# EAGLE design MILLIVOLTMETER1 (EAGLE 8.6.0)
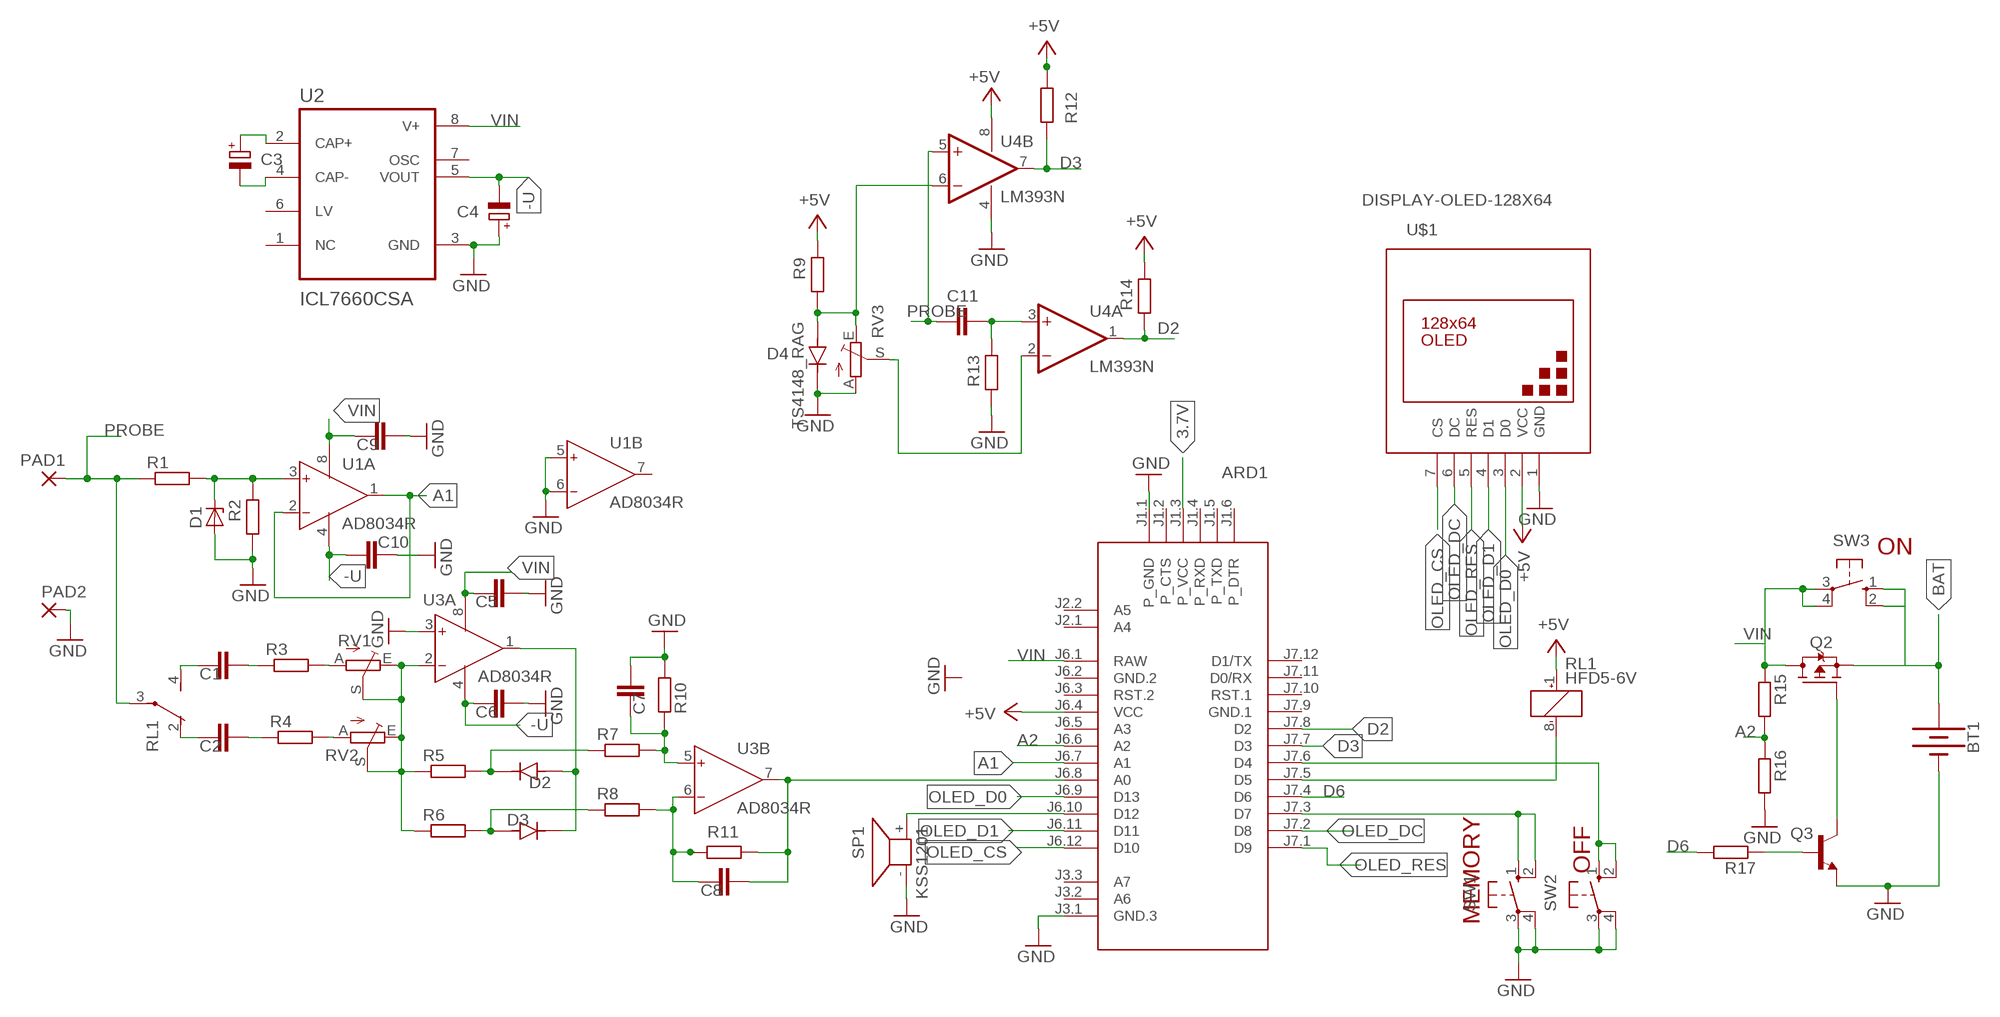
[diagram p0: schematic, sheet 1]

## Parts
ARD1  ARDUINO-PRO-MINI-3.3V  [ARDUINO-PRO-MINI]
BT1  BATTERY-9V  [BATTCON_9V]
C1  C-EUC0805  [C0805]
C2  C-EUC0805  [C0805]
C3  CPOL-EUSMCB  [SMC_B]
C4  CPOL-EUSMCB  [SMC_B]
C5  C-EUC0805  [C0805]
C6  C-EUC0805  [C0805]
C7  C-EUC0805  [C0805]
C8  C-EUC0805  [C0805]
C9  C-EUC0805  [C0805]
C10  C-EUC0805  [C0805]
C11  C-EUC0805  [C0805]
D1  ZENER-DIODESOD80C  [SOD80C]
D2  TS4148_RAG  [DIO_TS4148_RAG]
D3  TS4148_RAG  [DIO_TS4148_RAG]
D4  TS4148_RAG  [DIO_TS4148_RAG]
PAD1  3,81/1,1  [3,81/1,1]
PAD2  3,81/1,1  [3,81/1,1]
Q2  STR2P3LLH6  [SOT23]
Q3  BC817-16LT1SMD  [SOT23-BEC]
R1  R-EU_R0805  [R0805]
R2  R-EU_R0805  [R0805]
R3  R-EU_R0805  [R0805]
R4  R-EU_R0805  [R0805]
R5  R-EU_R0805  [R0805]
R6  R-EU_R0805  [R0805]
R7  R-EU_R0805  [R0805]
R8  R-EU_R0805  [R0805]
R9  R-EU_R0805  [R0805]
R10  R-EU_R0805  [R0805]
R11  R-EU_R0805  [R0805]
R12  R-EU_R0805  [R0805]
R13  R-EU_R0805  [R0805]
R14  R-EU_R0805  [R0805]
R15  R-EU_R0805  [R0805]
R16  R-EU_R0805  [R0805]
R17  R-EU_R0805  [R0805]
RL1  HFD5-6V  G6J-2P-Y  [G6J-2P-Y]
RV1  TRIM_EU-B64Y  [B64Y]
RV2  TRIM_EU-B64Y  [B64Y]
RV3  TRIM_EU-B64Y  [B64Y]
SP1  KSS1201  [KSS1201]
SW1  10-XX  [B3F-10XX]
SW2  10-XX  [B3F-10XX]
SW3  10-XX  [B3F-10XX]
U1  AD8034R  AD8033R  [SO8]
U2  ICL7660CSA  [SOIC127P600X175-8N]
U3  AD8034R  AD8033R  [SO8]
U4  LM393N  [DIL08]
U$1  DISPLAY-OLED-128X64  [DISPLAY-OLED-128X64]

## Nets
3.7V: ARD1.J1.3(P_VCC)
+5V: ARD1.J6.4(VCC) R9.1 R12.1 R14.1 RL1.1(1:+) U4.8(P:V+) U$1.2(VCC)
-U: C4.- C6.2 C10.2 U1.4(P:V-) U2.5(VOUT) U3.4(P:V-)
A1: ARD1.J6.7(A1) U1.1(A:OUT) U1.2(A:IN-)
A2: ARD1.J6.6(A2) R15.2 R16.1
BAT: BT1.+ Q2.3(S) SW3.1(S) SW3.2(S1)
D2: ARD1.J7.8(D2) R14.2 U4.1(A:OUT)
D3: ARD1.J7.7(D3) R12.2 U4.7(B:OUT)
D6: ARD1.J7.4(D6) R17.2
GND: ARD1.J1.1(P_GND) ARD1.J3.1(GND.3) BT1.- C4.+ C5.1 C6.1 C7.1 C9.1 C10.1 D1.A D4.C(K) PAD2.1(P) Q3.E R2.2 R10.1 R13.2 R16.2 RV3.A SP1.- SW1.3(P) SW1.4(P1) SW2.3(P) SW2.4(P1) U1.5(B:IN+) U1.6(B:IN-) U2.3(GND) U3.3(A:IN+) U4.4(P:V-) U$1.1(GND)
N$1: C1.2 RL1.4(2:S)
N$2: D1.C R1.2 R2.1 U1.3(A:IN+)
N$3: C11.1 R13.1 U4.3(A:+IN)
N$4: C3.+ U2.2(CAP+)
N$5: C3.- U2.4(CAP-)
N$6: ARD1.J7.3(D7) SW1.1(S) SW1.2(S1)
N$7: D4.A R9.2 RV3.E U4.6(B:-IN)
N$8: ARD1.J7.6(D4) SW2.1(S) SW2.2(S1)
N$9: ARD1.J6.10(D12) SP1.+
N$10: RV3.S U4.2(A:-IN)
N$11: C1.1 R3.1
N$12: C2.2 RL1.2(2:O)
N$13: C2.1 R4.1
N$14: R3.2 RV1.A
N$15: R4.2 RV2.A
N$16: Q2.2(G) Q3.C
N$17: R5.1 R6.1 RV1.E RV1.S RV2.E RV2.S U3.2(A:IN-)
N$18: Q3.B R17.1
N$19: D2.C(K) R5.2 R7.1
N$20: D3.A R6.2 R8.1
N$21: D2.A D3.C(K) U3.1(A:OUT)
N$22: C7.2 R7.2 R10.2 U3.5(B:IN+)
N$23: C8.2 R8.2 R11.1 U3.6(B:IN-)
N$24: ARD1.J6.8(A0) C8.1 R11.2 U3.7(B:OUT)
N$25: ARD1.J7.5(D5) RL1.8(1:-)
OLED_CS: ARD1.J6.12(D10) U$1.7(CS)
OLED_D0: ARD1.J6.9(D13) U$1.3(D0)
OLED_D1: ARD1.J6.11(D11) U$1.4(D1)
OLED_DC: ARD1.J7.2(D8) U$1.6(DC)
OLED_RES: ARD1.J7.1(D9) U$1.5(RES)
PROBE: C11.2 PAD1.1(P) R1.1 RL1.3(2:P) U4.5(B:+IN)
VIN: ARD1.J6.1(RAW) C5.2 C9.2 Q2.1(D) R15.1 SW3.3(P) SW3.4(P1) U1.8(P:V+) U2.8(V+) U3.8(P:V+)
Unconnected: ARD1.J1.2(P_CTS) ARD1.J1.4(P_RXD) ARD1.J1.5(P_TXD) ARD1.J1.6(P_DTR) ARD1.J2.1(A4) ARD1.J2.2(A5) ARD1.J3.2(A6) ARD1.J3.3(A7) ARD1.J6.3(RST.2) ARD1.J6.5(A3) ARD1.J7.10(RST.1) ARD1.J7.11(D0/RX) ARD1.J7.12(D1/TX) RL1.5(3:S) RL1.6(3:P) RL1.7(3:O) U1.7(B:OUT) U2.1(NC) U2.6(LV) U2.7(OSC)

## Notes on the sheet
- ON
- OFF
- MEMORY

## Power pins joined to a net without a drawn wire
GND.1: ARD1.J7.9(GND.1)
GND.2: ARD1.J6.2(GND.2)

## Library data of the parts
ARD1 = diy-modules:ARDUINO-PRO-MINI-*: Arduino Pro Mini and compatible devices More details available here: https://www.arduino.cc/en/Main/ArduinoBoardProMini Click here to find device on ebay.com
BT1 = SparkFun-Batteries:BATTERY: Battery - Single Cell; PROD_ID: BATT-10855
C1 C2 C5-C11 = rcl:C-EU: CAPACITOR, European symbol
C3 C4 = rcl:CPOL-EU: POLARIZED CAPACITOR, European symbol
D1 = diode:ZENER-DIODE: Z-Diode
D2-D4 = TS4148_RAG:TS4148_RAG: Check availability; AVAILABILITY: In Stock; CHECK_PRICES: https://www.snapeda.com/parts/TS4148%20RAG/Taiwan+Semiconductor/view-part/?ref=eda; DESCRIPTION: 1206 (Ceramics), 75V, 0.15A, Switching Diode & Array; MF: Taiwan Semiconductor; MP: TS4148 RAG; PACKAGE: 1206-2 Taiwan Semiconductor; PRICE: None; SNAPEDA_LINK: https://www.snapeda.com/parts/TS4148%20RAG/Taiwan+Semiconductor/view-part/?ref=snap
PAD1 PAD2 = wirepad:3,81/1,1: THROUGH-HOLE PAD
Q2 = transistor-fet:STR2P3LLH6
Q3 = transistor-npn:BC817*: NPN Transistor
R1-R17 = rcl:R-EU_: RESISTOR, European symbol
RL1 = relay:G6J*-2?-Y: Surface-Mounting Signal Relay - G6J-Y 5.7 x 10.6 x 9 mm Source: http://www.omroncomponents.eu/ .. K125-E2-02-X.pdf; MF: OMRON COMPONENTS USA; MPN: G6J-2P-Y-DC12; OC_FARNELL: unknown; OC_NEWARK: 70J9830
RV1-RV3 = pot:TRIM_EU-: POTENTIOMETER
SP1 = buzzer:KSS1201: SPEAKER; OC_FARNELL: unknown; OC_NEWARK: unknown
SW1-SW3 = switch-omron:10-XX: OMRON SWITCH; MPN: B3F-1000; OC_FARNELL: 176432; OC_NEWARK: 36M3542
U1 U3 = analog-devices:AD8033: 2.7 V, 800 ?A, 80 MHz Rail-to-Rail I/O Amplifiers Source: http://www.analog.com/static/imported-files/data_sheets/AD8031_8032.pdf; MF: ALTERA CORPORATION; MPN: AD8033ARZ; OC_FARNELL: 8621519; OC_NEWARK: 59K6245
U2 = ICL7660CSA:ICL7660CSA: Check availability; AVAILABILITY: In Stock; CHECK_PRICES: https://www.snapeda.com/parts/ICL7660CSA/Analog+Devices/view-part/?ref=eda; DESCRIPTION: Charge Pump Switching Regulator IC Positive or Negative Fixed -Vin, nVin, Vin/2 1 Output 20mA 8-SOIC (0.154, 3.90mm Width); MF: Analog Devices; MP: ICL7660CSA; PACKAGE: SOIC-8 Maxim; PRICE: None; SNAPEDA_LINK: https://www.snapeda.com/parts/ICL7660CSA/Analog+Devices/view-part/?ref=snap
U4 = linear:LM393: COMPARATOR
U$1 = diy-modules:DISPLAY-OLED-128X64: 128x64 Dot Matrix OLED Module based on SSD1306 chip Variant with SPI interface More details available here: http://www.instructables.com/id/How-to-use-OLED-display-arduino-module/ SSD1306 datasheet: https://cdn-shop.adafruit.com/datasheets/SSD1306.pdf Click here to find device on ebay.com Note: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

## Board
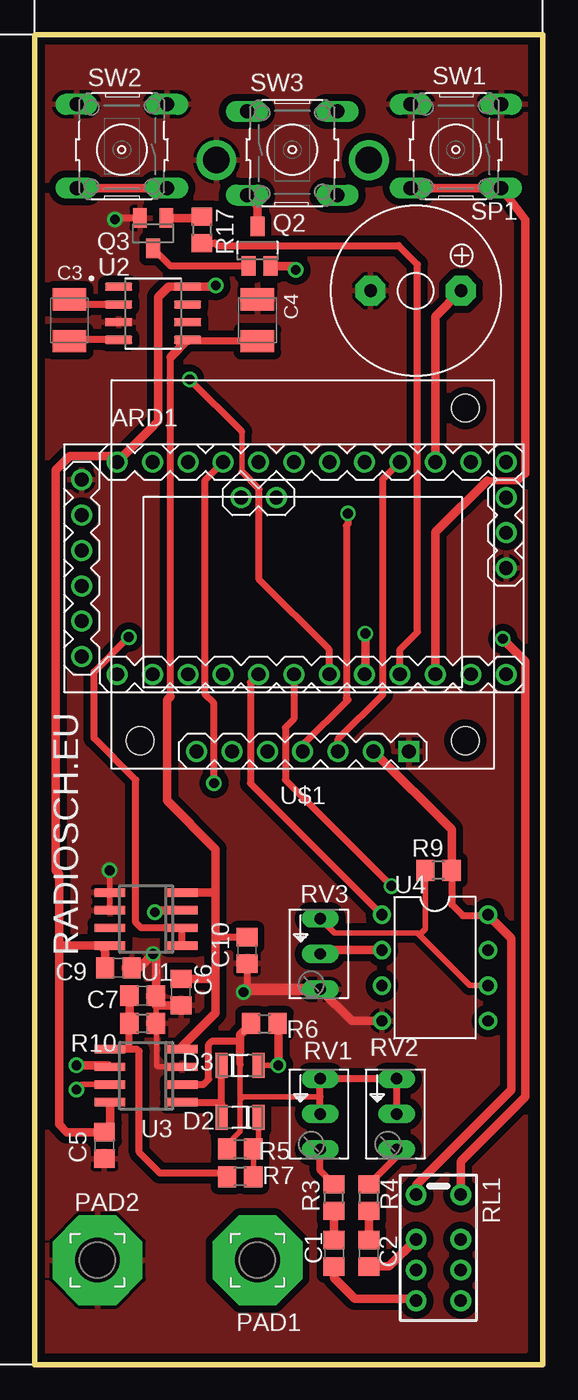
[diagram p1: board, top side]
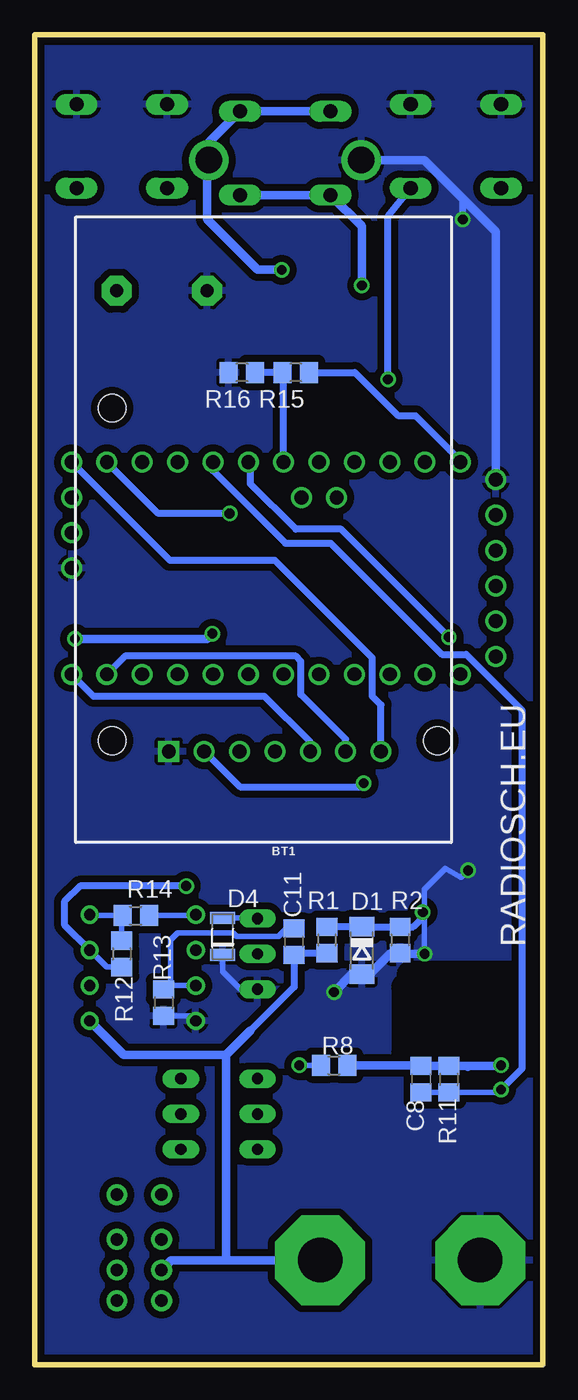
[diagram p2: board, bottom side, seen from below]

Size 36.5 x 95.5 mm. Coordinates in mm from the lower left corner, seen from the top.
Outline: 0,0 36.5,0 36.5,95.5 0,95.5 0,0
Copper layers (1*16): Top 0.035mm / dielectric 1.5mm / Bottom 0.035mm
Design rules "default *": minimum track width 10mil, minimum drill 24mil, track to track 8mil, track to pad 8mil, pad to pad 8mil, via to via 8mil, smd to smd 8mil, copper to edge 20mil, drill to drill 8mil, minimum pad ring 10mil, minimum via ring 8mil, stop-mask expansion 4mil, vias tented up to drill 0mil, thermal gap 10mil
bRestrict: area 0.2,22.4 to 9.9,28

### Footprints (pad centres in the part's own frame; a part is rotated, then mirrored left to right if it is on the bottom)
ARDUINO-PRO-MINI = drill 1: J1.1 -15.24,6.35; J1.2 -15.24,3.81; J1.3 -15.24,1.27; J1.4 -15.24,-1.27; J1.5 -15.24,-3.81; J1.6 -15.24,-6.35; J2.1 -1.27,5.08; J2.2 -3.81,5.08; J3.1 15.24,0; J3.2 15.24,2.54; J3.3 15.24,5.08; J6.1 -12.7,7.62; J6.2 -10.16,7.62; J6.3 -7.62,7.62; J6.4 -5.08,7.62; J6.5 -2.54,7.62; J6.6 0,7.62; J6.7 2.54,7.62; J6.8 5.08,7.62; J6.9 7.62,7.62; J6.10 10.16,7.62; J6.11 12.7,7.62; J6.12 15.24,7.62; J7.1 15.24,-7.62; J7.2 12.7,-7.62; J7.3 10.16,-7.62; J7.4 7.62,-7.62; J7.5 5.08,-7.62; J7.6 2.54,-7.62; J7.7 0,-7.62; J7.8 -2.54,-7.62; J7.9 -5.08,-7.62; J7.10 -7.62,-7.62; J7.11 -10.16,-7.62; J7.12 -12.7,-7.62
BATTCON_9V = drill 1.905: + -4,-1; - -4,-11.954
C0805 = smd 1.3 x 1.5: 1 -0.95,0; 2 0.95,0
SMC_B = smd 1.6 x 2.4: + -1.5,0; - 1.5,0
SOD80C = smd 1.4 x 1.8: A 1.7,0; C -1.7,0
DIO_TS4148_RAG = smd 0.85 x 1.8: A 1.325,0; C -1.325,0
3,81/1,1 = drill 3.2 pad 6.452 octagon: 1 0,0
SOT23 = smd 1 x 1.4: 1 0,1.735; 2 -0.632,-1.1; 3 0.95,-1.1
SOT23-BEC = smd 1 x 1.4: B -0.95,-1.1; C 0,1.1; E 0.95,-1.1
R0805 = smd 1.3 x 1.5: 1 -0.95,0; 2 0.95,0
G6J-2P-Y = drill 0.9 pad 1.5: 1 -3.2,-1.6; 2 0,-1.6; 3 2.2,-1.6; 4 4.4,-1.6; 5 4.4,1.6; 6 2.2,1.6; 7 0,1.6; 8 -3.2,1.6
B64Y = drill 0.813 long: A 2.54,0; E -2.54,0; S 0,0
KSS1201 = drill 0.914 pad 2.159 octagon: + 3.251,0; - -3.251,0
B3F-10XX = drill 1.016 long: 1 -3.251,2.761; 2 3.251,2.761; 3 -3.251,-3.261; 4 3.251,-3.261
SO8 = smd 0.6 x 2.2: 1 -1.905,-2.6; 2 -0.635,-2.6; 3 0.635,-2.6; 4 1.905,-2.6; 5 1.905,2.6; 6 0.635,2.6; 7 -0.635,2.6; 8 -1.905,2.6
SOIC127P600X175-8N = smd 1.97 x 0.59: 1 -2.475,1.905; 2 -2.475,0.635; 3 -2.475,-0.635; 4 -2.475,-1.905; 5 2.475,-1.905; 6 2.475,-0.635; 7 2.475,0.635; 8 2.475,1.905
DIL08 = drill 0.813 pad 1.27: 1 -3.81,-3.81; 2 -1.27,-3.81; 3 1.27,-3.81; 4 3.81,-3.81; 5 3.81,3.81; 6 1.27,3.81; 7 -1.27,3.81; 8 -3.81,3.81
DISPLAY-OLED-128X64 = drill 1 square: 1 -7.62,12.7 | drill 1: 2 -5.08,12.7; 3 -2.54,12.7; 4 0,12.7; 5 2.54,12.7; 6 5.08,12.7; 7 7.62,12.7 | hole 2: -11.684,11.938; 11.684,11.938; -11.684,-11.938

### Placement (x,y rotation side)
ARD1  18.62,57.2 0 top
BT1  25,90.5 90 bottom
C1  21.5,8 270 top
C2  24,8 270 top
C3  2.5,75 270 top
C4  16,75 270 top
C5  5,15.75 90 top
C6  10.5,26.75 90 top
C7  7.75,26.5 180 top
C8  8.75,20.5 90 bottom
C9  6,28.5 180 top
C10  15.25,29.75 90 top
C11  17.88,30.38 270 bottom
D1  13,29.75 270 bottom
D2  14.75,17.75 180 top
D3  14.75,21.5 0 top
D4  23,30.75 90 bottom
PAD1  16,7.5 0 top
PAD2  4.5,7.5 0 top
Q2  16,80 0 top
Q3  8.5,81.25 180 top
R1  15.5,30.5 90 bottom
R2  10.25,30.5 270 bottom
R3  21.5,12 90 top
R4  24,12 90 top
R5  14.75,15.5 0 top
R6  16.5,24.5 0 top
R7  14.75,13.5 180 top
R8  15,21.5 0 bottom
R9  29,35.5 180 top
R10  7.75,24.5 180 top
R11  6.75,20.5 270 bottom
R12  30.25,29.5 270 bottom
R13  27.25,26 270 bottom
R14  29.25,32.25 0 bottom
R15  17.75,71.25 180 bottom
R16  21.62,71.25 180 bottom
R17  12,81.5 270 top
RL1  29,9 270 top
RV1  20.5,18 270 top
RV2  26,18 270 top
RV3  20.5,29.5 270 top
SP1  27.38,77.12 0 top
SW1  30.25,87.25 180 top
SW2  6.25,87.25 180 top
SW3  18.5,87.25 0 top
U1  8,32 90 top
U2  8.5,75.5 0 top
U3  8,20.75 90 top
U4  28.75,28.5 270 top
U$1  19.25,56.75 180 top

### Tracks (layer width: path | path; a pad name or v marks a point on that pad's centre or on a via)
+5V  (via drill 0.7)
  Top 0.5: R9.1 29.95,33.05 30.75,32.25 32.5,32.25 U4.8 | v12.88,41.75 12.88,47.5 12.25,48.12 12.25,63.53 ARD1.J6.4
  Top 0.61: RL1.1 27.4,12.9 34.25,19.75 34.25,30.62 U4.8 | R9.1 29.95,38.43 U$1.2
  Bottom 0.406: U4.8 32.5,32.25 R14.1 30.25,32.2 R12.1
  Bottom 0.5: U$1.2 24.3,44.05 21.75,41.5 13.12,41.5 v12.88,41.75
-U
  Top 0.5: C10.2 13.3,30.7 13,31 | C4.- 11.07,73.5 U2.5 | 9.75,48 9.75,72.37
  Top 0.61: U3.4 10.6,22.85 13,25.25 13,27.5 | 13,27.5 13,31 13,34 | U1.4 12.9,33.91 13,34 | C6.2 12.8,27.7 13,27.5 | 13,34 13,37 9.5,40.5 9.5,47.75 9.75,48 | 9.75,72.37 U2.5
A1  (via drill 0.7)
  Top 0.5: U1.1 U1.2 7.63,31.36 7.25,31.75 7.25,42 4.25,45 4.25,49.75 v6.75,52.25
  Bottom 0.5: v6.75,52.25 14.5,60 17.75,60 21,63.25 21,64.66 ARD1.J6.7
A2
  Bottom 0.5: ARD1.J6.6 18.62,71.17 R15.2 R16.1
BAT  (via drill 0.7)
  Top 0.61: Q2.3 18.48,78.9 v18.75,78.62
  Bottom 0.61: SW3.1 SW3.2 24,87.76 BT1.+ 24.12,86.38 24.12,82.25 20.5,78.62 v18.75,78.62
D2
  Top 0.5: U4.1 15.5,41.75 15.5,49 ARD1.J7.8
  Bottom 0.406: R14.2 25,32.25 U4.1
D3  (via drill 0.7)
  Top 0.5: ARD1.J7.7 18.62,46.37 18,45.75 18,42 v25.62,34.38
  Bottom 0.406: R12.2 31.34,28.55 U4.7
  Bottom 0.5: v25.62,34.38 33.25,34.38 34.38,33.25 34.38,31.59 U4.7
D6
  Top 0.5: R17.2 12.95,80.55 13.12,80.38 26.12,80.38 27.5,79 27.5,52.62 26.24,51.37 ARD1.J7.4
GND  (via drill 0.7)
  Top 0.406: U3.3 8.87,21.39 8.75,21.5 8.75,24.45 R10.1 8.7,25.75 C7.1 | U1.6 5.38,32.63 v5.38,35.5
  Top 0.5: C10.1 15.25,27 v15,26.75 | 21.29,27 RV3.A | Q3.E 5.85,82.35 v5.75,82.25
  Top 0.61: 8.75,24.55 R10.1 | C6.1 8.75,25.8 8.7,25.75 | U4.4 22.77,24.69 RV3.A | C9.1 7.5,28.5 v8.5,29.5 8.7,29.3 C7.1
  Top 0.813: RV3.A 15.21,26.96 v15,26.75
  Bottom 0.406: 21.29,27 21.75,27 23,28.25 D4.C | R13.2 25.3,25.05 U4.4 | v5.38,35.5 5.88,35 7,35.62 8.5,34.12 v8.5,29.5
  Bottom 0.5: 21.29,27 RV3.A | v5.75,82.25 5.75,83.75 5.88,83.87
  Bottom 0.61: v15,26.75 13.7,28.05 D1.A 12.95,28 12.5,28 10.95,29.55 R2.2 10.2,29.5 v8.5,29.5 | ARD1.J1.1 3.38,81.38 5.88,83.87 8.51,86.5 BT1.-
  pour Top (isolate 0.5): 0.5,95 35.25,95 35.25,1 0.5,1
  pour Bottom (isolate 0.5): 0.5,94.75 35.75,94.75 35.75,0.5 0.5,0.5
N$1
  Top 0.61: C1.2 21.5,6.25 23,4.75 27.25,4.75 RL1.4
N$2  (via drill 0.7)
  Top 0.61: U1.3 8.76,32.63 v8.62,32.5
  Bottom 0.5: R1.2 D1.C R2.1 9.3,31.45 8.62,32.12 v8.62,32.5
N$3
  Bottom 0.406: C11.1 17.95,31.25 18.5,31.25 19,30.75 22,30.75 22.25,31 26.25,31 26.75,30.5 26.75,27.45 | 26.75,27.45 R13.1 | U4.3 26.53,27.23 26.75,27.45
N$4
  Top 0.5: U2.2 2.87,76.14 C3.+
N$5
  Top 0.5: U2.4 2.6,73.59 C3.-
N$6
  Top 0.5: 32.5,63.5 34.75,63.5 35.25,64
  Top 0.61: ARD1.J7.3 28.78,59.78 32.5,63.5 | SW1.2 SW1.1 35.25,82.24 35.25,64
N$7
  Top 0.406: U4.6 31.27,27.23 27.62,30.88 | 27.62,30.88 27.5,31 21.54,31 RV3.E | R9.2 28.05,31.3 27.62,30.88
  Bottom 0.406: D4.A 20.54,32.08 RV3.E
N$8  (via drill 0.7)
  Top 0.406: 14.88,64.12 14.88,67
  Top 0.5: ARD1.J7.6 21.16,51.34 16.12,56.38 16.12,62.88 14.88,64.12 | 14.88,67 v11.12,70.75
  Top 0.61: SW2.2 SW2.1
  Bottom 0.5: v11.12,70.75 11.12,82.49 SW2.1
N$9
  Top 0.61: ARD1.J6.10 28.78,75.28 SP1.+
N$10
  Top 0.61: U4.2 20.77,29.77 RV3.S
N$11
  Top 0.61: C1.1 R3.1
N$12
  Top 0.61: C2.2 25.45,7.05 RL1.2
N$13
  Top 0.61: C2.1 R4.1
N$14
  Top 0.5: R3.2 20.5,13.95 RV1.A
N$15
  Top 0.5: R4.2 26,14.95 RV2.A
N$16
  Top 0.5: Q2.2 9.75,78.9 Q3.C
N$17
  Top 0.406: 14.75,21.55 14.75,19.25 15,19.25 | 20.5,19.25 15,19.25 | R5.1 13.8,15.8 14.75,16.75 14.75,19 15,19.25
  Top 0.5: RV1.S 20.5,19.25 RV1.E RV2.E RV2.S | 14.75,21.55 14.75,22.5 | U3.2 12.12,20.11 12.5,20.5 12.5,23 12.75,23.25 14.75,23.25
  Top 0.61: 14.75,22.5 14.75,23.25 14.75,23.7 R6.1
N$18
  Top 0.61: Q3.B 11.9,82.35 R17.1
N$19
  Top 0.406: R7.1 R5.2 16.07,15.88 D2.C
N$20  (via drill 0.7)
  Top 0.406: v17.5,21.5 D3.A
  Top 0.61: v17.5,21.5 17.5,24.45 R6.2
  Bottom 0.406: R8.1 v17.5,21.5
N$21
  Top 0.5: D2.A 13.43,18.75 | 13.43,18.75 D3.C | U3.1 13.33,18.84 13.43,18.75
N$22
  Top 0.5: R7.2 13.55,13.75 9,13.75 7.5,15.25 7.5,22.5 7.34,22.66 6.75,22.66 | 6.75,22.66 U3.5 | R10.2 6.75,24.45 6.75,22.66
  Top 0.61: R10.2 C7.2
N$23  (via drill 0.7)
  Top 0.61: v3,21.5 5.29,21.5 U3.6
  Bottom 0.61: R8.2 8.75,21.5 C8.2 R11.1 | R11.1 3.05,21.45 v3,21.5 | R11.1 5.46,21.45 U3.6
N$24  (via drill 0.7)
  Top 0.406: U3.7 3.37,20.11 v3,19.75
  Bottom 0.406: v3,19.75 3.2,19.55 R11.2 C8.1
  Bottom 0.5: v3,19.75 1.5,21.25 1.5,47 5.5,51 7.25,51 15.25,59 18.5,59 23.7,64.2 ARD1.J6.8
N$25  (via drill 0.7)
  Top 0.61: RL1.8 30.6,14.6 35.25,19.25 35.25,50.5 v33.62,52.12 | v23.75,52.5 23.75,49.63 ARD1.J7.5
  Bottom 0.61: v33.62,52.12 24.12,52.12 v23.75,52.5
OLED_CS
  Bottom 0.5: U$1.7 11.63,47.38 12.25,48 12.25,50.75 19.25,57.75 26.79,57.75 ARD1.J6.12
OLED_D0
  Top 0.5: U$1.3 21.79,44.91 25,48.12 25,63.58 ARD1.J6.9
OLED_D1  (via drill 0.7)
  Top 0.5: U$1.4 19.25,44.5 22.5,47.75 22.38,47.88 22.38,60.25 22.5,60.38 v22.5,61.12
  Bottom 0.5: v22.5,61.12 27.62,61.12 ARD1.J6.11
OLED_DC
  Bottom 0.5: U$1.6 14.17,44.92 17.38,48.12 17.38,50.5 17.75,50.88 30.02,50.88 ARD1.J7.2
OLED_RES
  Bottom 0.5: U$1.5 16.71,44.71 20,48 32.28,48 ARD1.J7.1
PROBE
  Bottom 0.5: R1.1 17.75,29.55 C11.2 17.88,27.12 21,24
  Bottom 0.61: PAD1.1 22.75,7.5 | 22.75,7.5 26.7,7.5 RL1.3 | 21,24 22.75,22.25 | 22.75,22.25 22.75,7.5 | 22.75,22.25 30.12,22.25 U4.5
VIN  (via drill 0.7)
  Top 0.61: U3.8 5.4,17.1 C5.2 2.3,16.7 1.75,17.25 1.75,29.75 | 1.75,29.75 1.75,35.25 1.5,35.5 1.5,64.25 2.5,65.25 5.49,65.25 ARD1.J6.1 8.25,67.15 8.28,67.15 8.88,67.75 8.88,76.66 9.62,77.41 U2.8 12.9,77.41 v13,77.5 | U1.8 4.75,30.09 | 4.75,30.09 2.1,30.09 1.75,29.75 | C9.2 5.05,29.8 4.75,30.09 | Q2.1 16,83.24 SW3.3
  Bottom 0.5: R15.1 13.5,71.25 10.38,68.12 9.12,68.12 5.92,64.92 ARD1.J6.1
  Bottom 0.61: SW3.4 SW3.3 13,81.74 v13,77.5

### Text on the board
tPlace: RADIOSCH.EU
bPlace: RADIOSCH.EU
